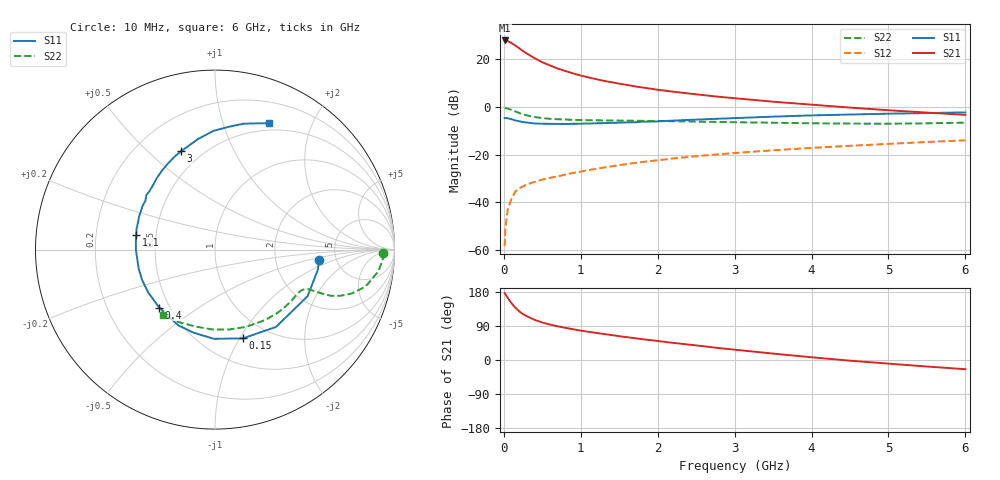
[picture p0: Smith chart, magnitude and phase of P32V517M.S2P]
! SIEMENS Small Signal Semiconductors
! BFP181
! Si NPN RF Bipolar Junction Transistor in SOT143
! VCE = 2.5 V  IC = 17 mA
! Common Emitter S-Parameters:  March  1996
# GHz  S  MA  R  50
!  f  S11  S21  S12  S22
! GHz  MAG  ANG  MAG  ANG  MAG  ANG  MAG  ANG
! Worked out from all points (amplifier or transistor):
!   36 points, 10 MHz to 6 GHz, reference 50 ohm
!   highest |S21| = 27.8 dB at 10 MHz (marker M1)
!   |S21| within 3 dB of that: start of sweep to 187.9 MHz
!   unconditionally stable (mu >= 1): start of sweep to 12.99 MHz; 527.7 MHz to end of sweep
!   at 250 MHz: K = 0.62, MSG = 28.4 dB, |S12| = -33.4 dB
!   at 1.4 GHz: K = 1.41, MAG = 13.8 dB, |S12| = -25.0 dB
!   at 6 GHz: K = 1.10, MAG = 3.4 dB, |S12| = -14.0 dB
!   S11 on the Smith chart (normalised r, x): 10 MHz: 3.65, -0.63; 150 MHz: 0.76, -1.03; 400 MHz: 0.44, -0.35; 1.1 GHz: 0.38, +0.08; 3 GHz: 0.39, +0.64; 6 GHz: 0.42, +1.43
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0.01  0.5802 -5.7  24.61 176.6  0.0012 86.4  0.9382 -1.2
0.02  0.5845 -10.9  24.57 173.8  0.0028 79.9  0.9384 -2.9
0.05  0.5773 -26.8  23.91 164.0  0.0069 80.2  0.9181 -7.6
0.1  0.5487 -51.8  21.68 149.8  0.0119 66.8  0.8647 -13.7
0.15  0.5183 -72.6  19.26 138.0  0.0167 61.6  0.8003 -17.8
0.2  0.4972 -90.7  16.87 128.5  0.0195 57.0  0.7427 -20.3
0.25  0.4781 -104.5  14.73 121.0  0.0215 53.0  0.696 -21.7
0.3  0.469 -115.9  13.08 115.5  0.0238 52.4  0.6604 -22.2
0.4  0.4481 -133.9  10.47 105.9  0.0267 50.9  0.6115 -22.6
0.5  0.4421 -147.3  8.6 99.0  0.0298 50.4  0.5804 -22.8
0.6  0.44 -157.6  7.36 93.5  0.0325 51.4  0.5614 -23.1
0.7  0.4382 -165.8  6.341 88.9  0.0348 52.2  0.5497 -23.7
0.9  0.4408 179.9  5.03 81.2  0.0412 53.9  0.534 -25.0
1.1  0.4474 169.4  4.144 74.4  0.0475 54.4  0.5247 -27.0
1.5  0.4645 153.0  3.064 62.8  0.0599 55.2  0.5145 -32.1
1.8  0.4889 141.4  2.546 54.9  0.0697 54.5  0.5078 -36.5
2.2  0.5139 129.1  2.079 45.2  0.0828 52.6  0.4986 -43.0
3  0.5797 109.0  1.516 27.3  0.1076 47.6  0.4754 -57.6
3.5  0.6228 98.8  1.281 16.9  0.1229 44.1  0.4641 -68.1
4.5  0.6894 83.4  0.963 -1.8  0.1524 36.1  0.4453 -91.8
5.5  0.7395 72.0  0.757 -17.2  0.1833 28.3  0.4512 -116.4
6  0.7645 67.0  0.678 -24.3  0.1986 23.9  0.4667 -128.5
